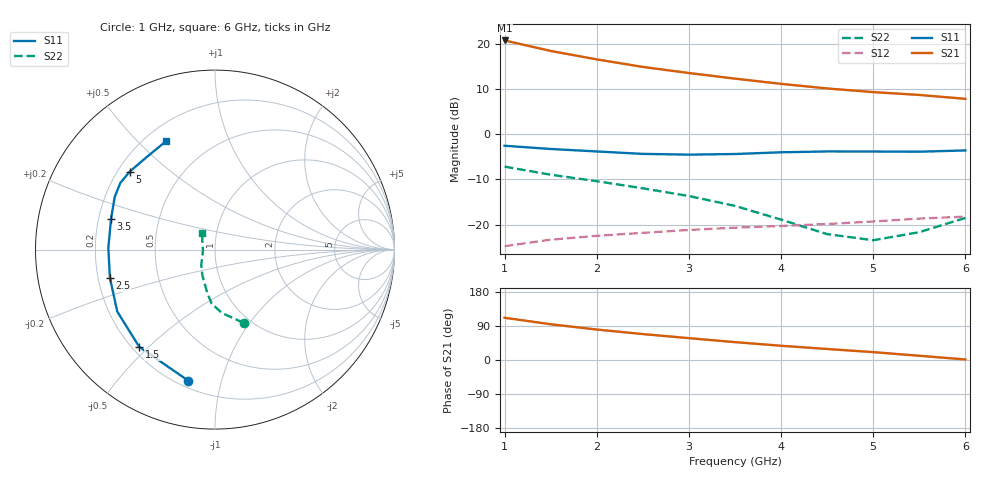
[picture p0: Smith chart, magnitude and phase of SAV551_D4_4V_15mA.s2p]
! Created Mon Oct 27 14:31:22 2008
# hz S ma R 50
! 2 Port Network Data from SP1.SP block
! freq  magS11  angS11  magS21  angS21  magS12  angS12  magS22  angS22
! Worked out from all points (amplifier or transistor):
!   11 points, 1 GHz to 6 GHz, reference 50 ohm
!   highest |S21| = 20.8 dB at 1 GHz (marker M1)
!   |S21| within 3 dB of that: start of sweep to 1.682 GHz
!   unconditionally stable (mu >= 1): 4.338 GHz to end of sweep
!   at 1.5 GHz: K = 0.47, MSG = 20.9 dB, |S12| = -23.3 dB
!   at 3.5 GHz: K = 0.91, MSG = 16.5 dB, |S12| = -20.7 dB
!   at 6 GHz: K = 1.10, MAG = 11.1 dB, |S12| = -18.2 dB
!   S11 on the Smith chart (normalised r, x): 1 GHz: 0.24, -0.79; 1.5 GHz: 0.23, -0.47; 2.5 GHz: 0.25, -0.12; 3.5 GHz: 0.25, +0.14; 5 GHz: 0.25, +0.37; 6 GHz: 0.28, +0.61
1e9  0.7457 -101.5  10.91 111.5  0.05773 39.3  0.438 -68.7
1.5e9  0.6868 -127.9  8.349 94.3  0.06811 30.6  0.3565 -83.5
2e9  0.6447 -147.7  6.734 80.4  0.07516 24.8  0.3022 -93.4
2.5e9  0.6062 -165.0  5.558 68.4  0.08106 20.5  0.2521 -99.3
3e9  0.5944 179.0  4.758 57.6  0.08727 17.3  0.2072 -105.3
3.5e9  0.6042 163.4  4.123 47.1  0.09251 13.1  0.1611 -115.9
4e9  0.6314 152.2  3.61 37.6  0.09648 9.8  0.1135 -132.5
4.5e9  0.6451 144.9  3.21 29.0  0.1016 7.8  0.07847 -153.0
5e9  0.6439 137.7  2.926 20.8  0.1083 4.9  0.06714 179.0
5.5e9  0.6408 126.5  2.722 11.2  0.1166 0.7  0.08245 148.8
6e9  0.662 114.5  2.464 1.4  0.1225 -4.0  0.1187 126.9
